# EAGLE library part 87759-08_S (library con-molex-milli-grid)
HEADER
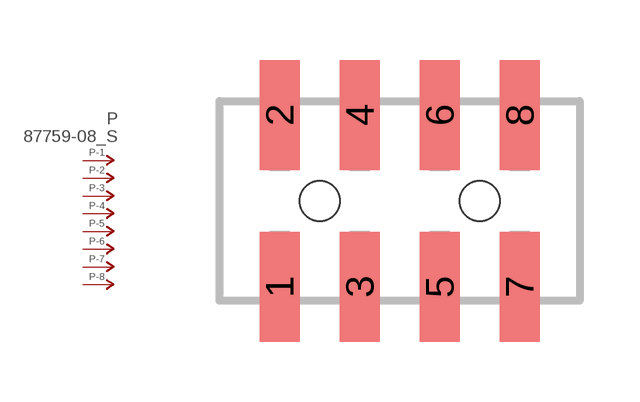
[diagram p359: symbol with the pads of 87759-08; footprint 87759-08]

Designator prefix P; gates -1=P-NV -2=P-N -3=P-N -4=P-N -5=P-N -6=P-N -7=P-N -8=P-N

## 87759-08_S  [87759-08]
1  -1:P  pas
2  -2:P  pas
3  -3:P  pas
4  -4:P  pas
5  -5:P  pas
6  -6:P  pas
7  -7:P  pas
8  -8:P  pas

## Footprint 87759-08 (pad centres in mm)
HEADER SMD Dual Row, Vertical
smd 1 x 2.75: 1 -3,-2.15; 2 -3,2.15; 3 -1,-2.15; 4 -1,2.15; 5 1,-2.15; 6 1,2.15; 7 3,-2.15; 8 3,2.15
hole 1 at -2,0
hole 1 at 2,0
